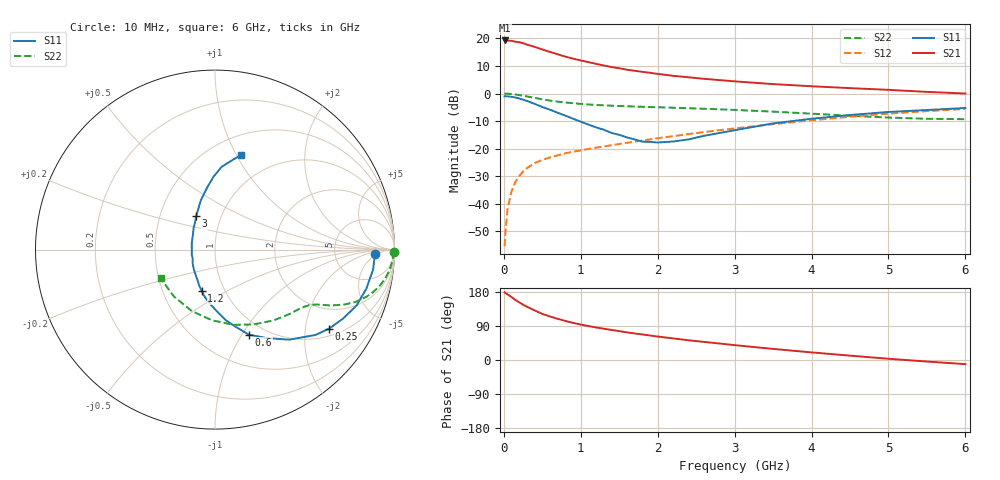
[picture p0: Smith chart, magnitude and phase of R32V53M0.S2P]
! SIEMENS Small Signal Semiconductors
! BFR181
! Si NPN RF Bipolar Junction Transistor in SOT23
! VCE = 2.5 V  IC = 3 mA
! Common Emitter S-Parameters:  May  1996
# GHz  S  MA  R  50
!  f  S11  S21  S12  S22
! GHz  MAG  ANG  MAG  ANG  MAG  ANG  MAG  ANG
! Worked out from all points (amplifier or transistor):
!   36 points, 10 MHz to 6 GHz, reference 50 ohm
!   highest |S21| = 19.2 dB at 10 MHz (marker M1)
!   |S21| within 3 dB of that: start of sweep to 471.5 MHz
!   unconditionally stable (mu >= 1): 1.341 GHz to 3.188 GHz
!   at 250 MHz: K = 0.30, MSG = 23.3 dB, |S12| = -28.3 dB
!   at 1.4 GHz: K = 1.01, MAG = 13.5 dB, |S12| = -18.8 dB
!   at 6 GHz: K = 0.86, MSG = 2.8 dB, |S12| = -5.6 dB
!   lowest NFmin = 1.40 dB at 450 MHz
!   S11 on the Smith chart (normalised r, x): 10 MHz: 16, -4; 250 MHz: 1.23, -2.70; 600 MHz: 0.84, -1.07; 1.2 GHz: 0.78, -0.38; 3 GHz: 0.76, +0.30; 6 GHz: 0.69, +1.04
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0.01  0.8901 -1.6  9.17 178.7  0.0017 94.5  0.9955 -0.7
0.02  0.8901 -2.8  8.987 176.9  0.003 87.1  0.9932 -1.4
0.05  0.8879 -7.2  9.114 172.9  0.0084 85.6  0.9908 -3.4
0.1  0.8706 -14.6  9.038 166.0  0.0167 82.3  0.9798 -6.7
0.15  0.848 -21.5  8.693 158.5  0.0248 77.7  0.9613 -9.8
0.2  0.8106 -28.3  8.528 152.1  0.0316 74.6  0.938 -12.6
0.25  0.7735 -34.7  8.188 145.9  0.0386 71.2  0.9116 -15.1
0.3  0.7341 -40.4  7.717 140.5  0.0442 69.0  0.8851 -17.2
0.4  0.6496 -50.6  7.023 130.9  0.0546 64.5  0.8346 -20.5
0.5  0.5692 -59.9  6.292 121.7  0.0624 61.6  0.7852 -22.9
0.6  0.5092 -68.4  5.68 114.8  0.0694 59.6  0.7436 -24.6
0.8  0.3964 -81.5  4.666 103.1  0.0824 57.7  0.6876 -26.7
0.9  0.3489 -87.5  4.294 98.0  0.088 57.7  0.6662 -27.5
1.1  0.2725 -101.6  3.705 89.6  0.0984 58.0  0.6327 -29.0
1.2  0.243 -107.7  3.454 85.8  0.104 58.2  0.6201 -29.8
1.6  0.1596 -138.1  2.701 72.9  0.1277 59.0  0.5879 -33.1
2.2  0.1347 164.3  2.094 57.0  0.1681 59.3  0.553 -40.0
3  0.2157 119.1  1.662 39.2  0.2325 56.7  0.5038 -52.2
3.5  0.2869 105.8  1.482 29.3  0.2777 53.6  0.469 -62.8
4.5  0.4069 91.1  1.252 11.5  0.3791 44.1  0.394 -92.5
5.5  0.5019 79.8  1.07 -4.1  0.4795 31.6  0.3474 -131.3
6  0.546 74.7  1 -10.9  0.5263 24.3  0.3425 -152.4
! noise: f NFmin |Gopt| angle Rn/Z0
0.45  1.4  0.56  17  0.36
0.9  1.5  0.45  35  0.34
1.8  1.85  0.25  82  0.36
